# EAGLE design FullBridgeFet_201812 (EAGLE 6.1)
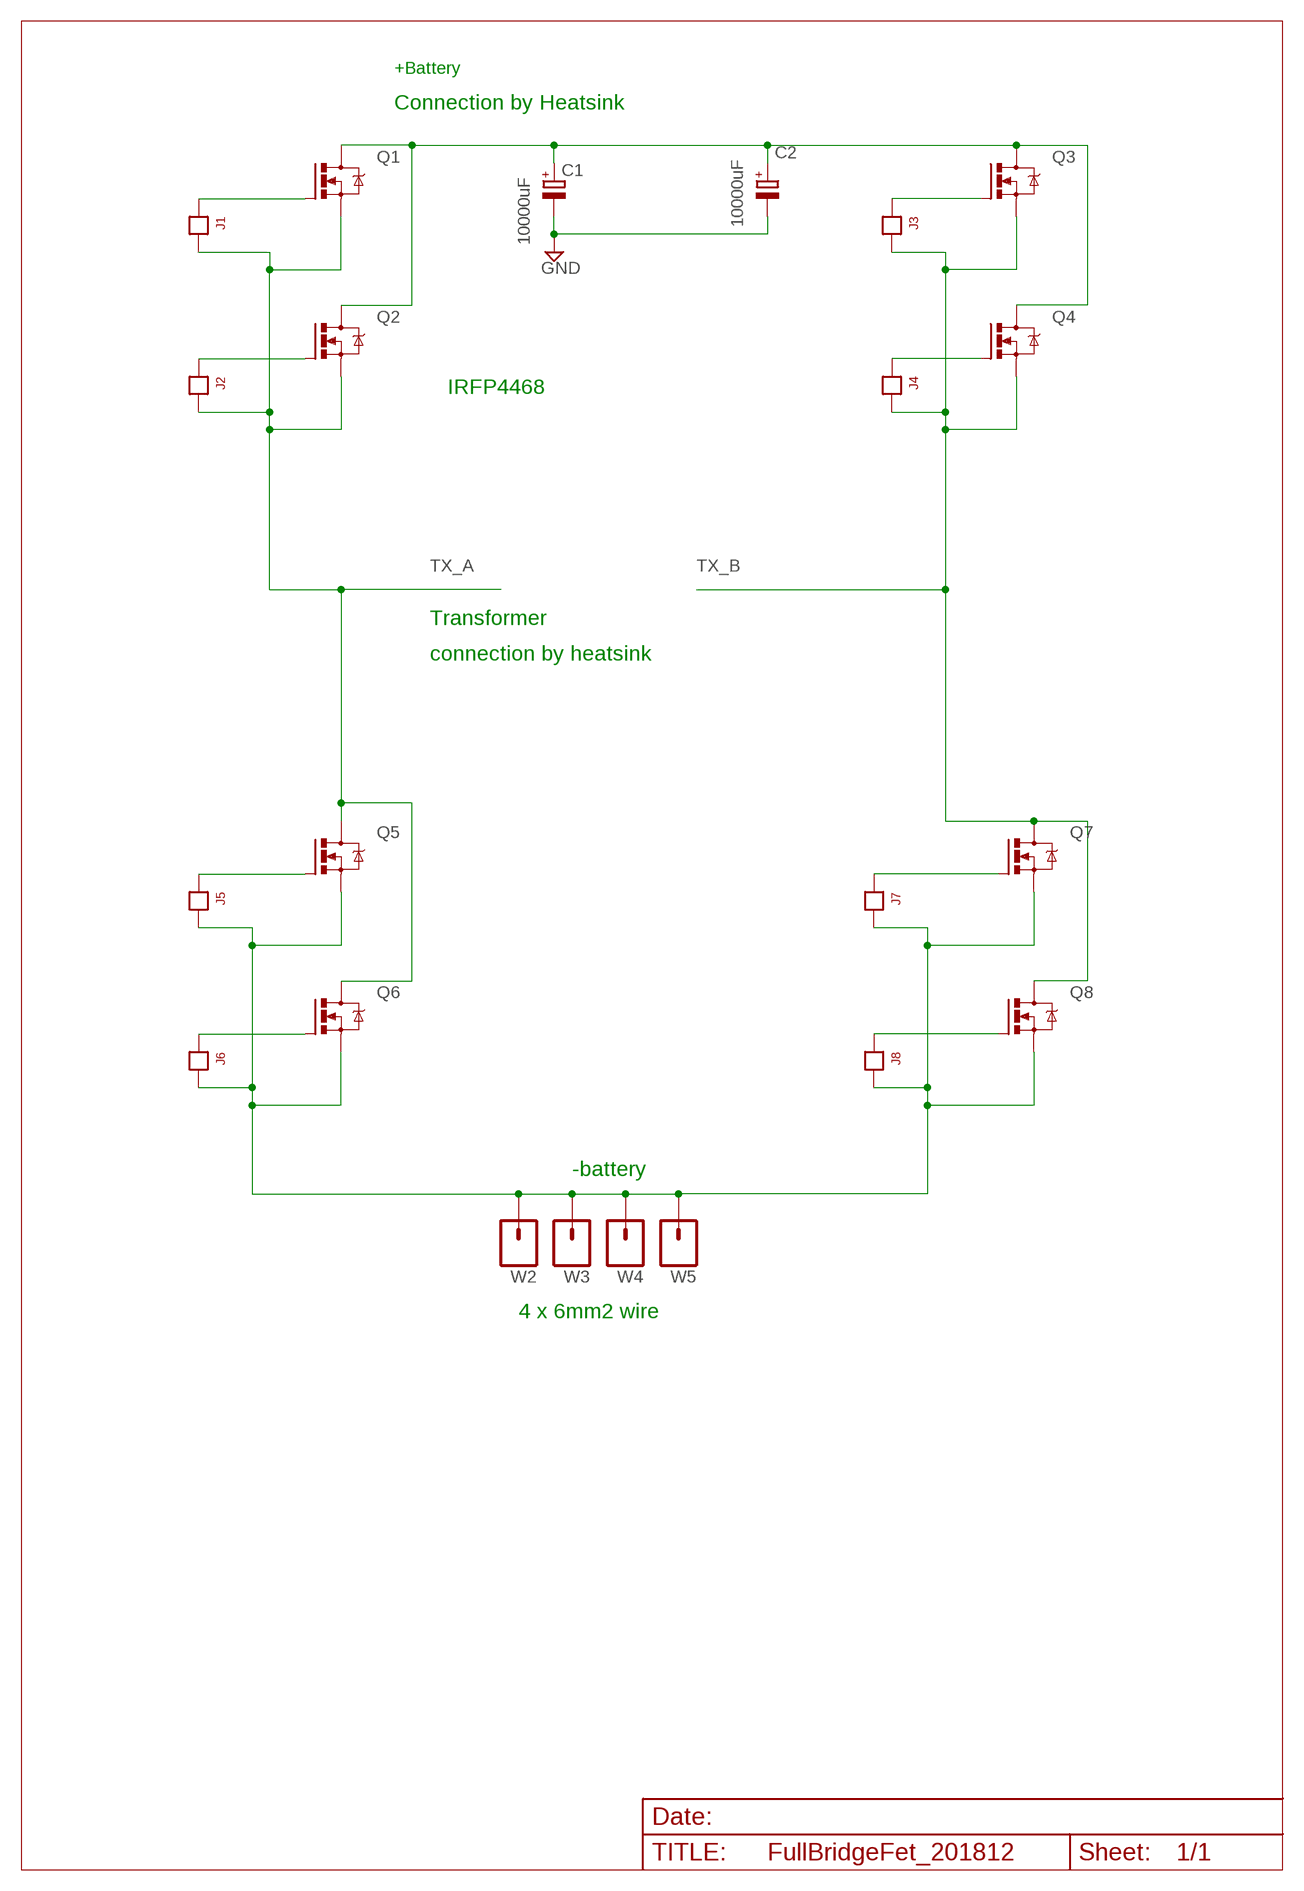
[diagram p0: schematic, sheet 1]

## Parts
C1  10000uF  C-RB3500LARGEPTH  [EB35D_LARGETH]
C2  10000uF  C-RB3500LARGEPTH  [EB35D_LARGETH]
J1  JP1  [JP1]
J2  JP1  [JP1]
J3  JP1  [JP1]
J4  JP1  [JP1]
J5  JP1  [JP1]
J6  JP1  [JP1]
J7  JP1  [JP1]
J8  JP1  [JP1]
Q1  IRFP4468  MOSFET-NCH-BIG  [TO247-WIRED]
Q2  MOSFET-NCH-BIG  [TO247-WIRED]
Q3  MOSFET-NCH-BIG  [TO247-WIRED]
Q4  MOSFET-NCH-BIG  [TO247-WIRED]
Q5  MOSFET-NCH-BIG  [TO247-WIRED]
Q6  MOSFET-NCH-BIG  [TO247-WIRED]
Q7  MOSFET-NCH-BIG  [TO247-WIRED]
Q8  MOSFET-NCH-BIG  [TO247-WIRED]
W2  M014MM2-WIREHOLE  [3.5MMWIREHOLE]
W3  M014MM2-WIREHOLE  [3.5MMWIREHOLE]
W4  M014MM2-WIREHOLE  [3.5MMWIREHOLE]
W5  M014MM2-WIREHOLE  [3.5MMWIREHOLE]

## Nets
+BATT: C1.+ C2.+ Q1.D Q1.DW(D) Q2.D Q2.DW(D) Q3.D Q3.DW(D) Q4.D Q4.DW(D)
GND: C1.- C2.- J5.2 J6.2 J7.2 J8.2 Q5.S Q5.SW(S) Q6.S Q6.SW(S) Q7.S Q7.SW(S) Q8.S Q8.SW(S) W2.P$1 W3.P$1 W4.P$1 W5.P$1
N$1: J1.1 Q1.G
N$2: J5.1 Q5.G
N$3: J6.1 Q6.G
N$4: J7.1 Q7.G
N$5: J2.1 Q2.G
N$6: J8.1 Q8.G
N$7: J3.1 Q3.G
N$10: J4.1 Q4.G
TX_A: J1.2 J2.2 Q1.S Q1.SW(S) Q2.S Q2.SW(S) Q5.D Q5.DW(D) Q6.D Q6.DW(D)
TX_B: J3.2 J4.2 Q3.S Q3.SW(S) Q4.S Q4.SW(S) Q7.D Q7.DW(D) Q8.D Q8.DW(D)

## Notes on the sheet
- +Battery
- Connection by Heatsink
- IRFP4468
- Transformer
- connection by heatsink
- -battery
- 4 x 6mm2 wire

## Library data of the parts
C1 C2 = Andrew Passive:C-RB3500
J1-J8 = Andrew Connectors:JP1
Q1-Q8 = Andrew Transistor:MOSFET-NCH-BIG
W2-W5 = Andrew:M01: Header 1

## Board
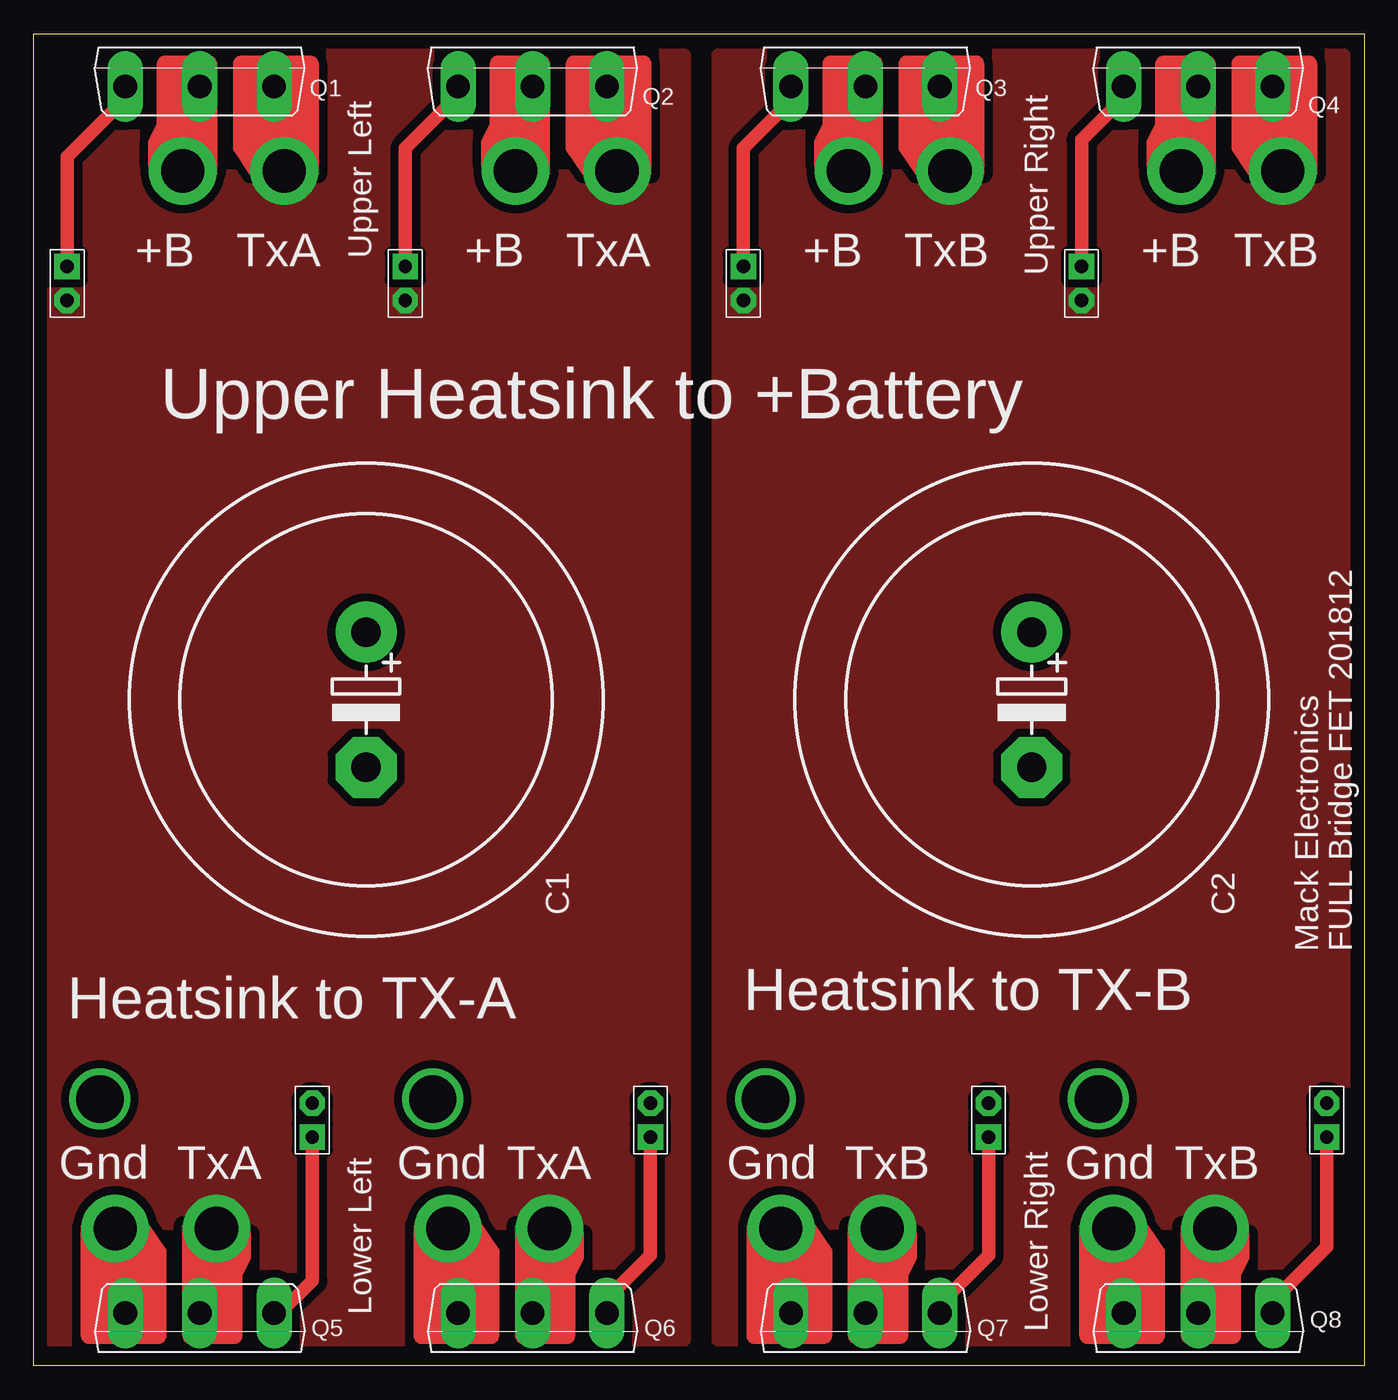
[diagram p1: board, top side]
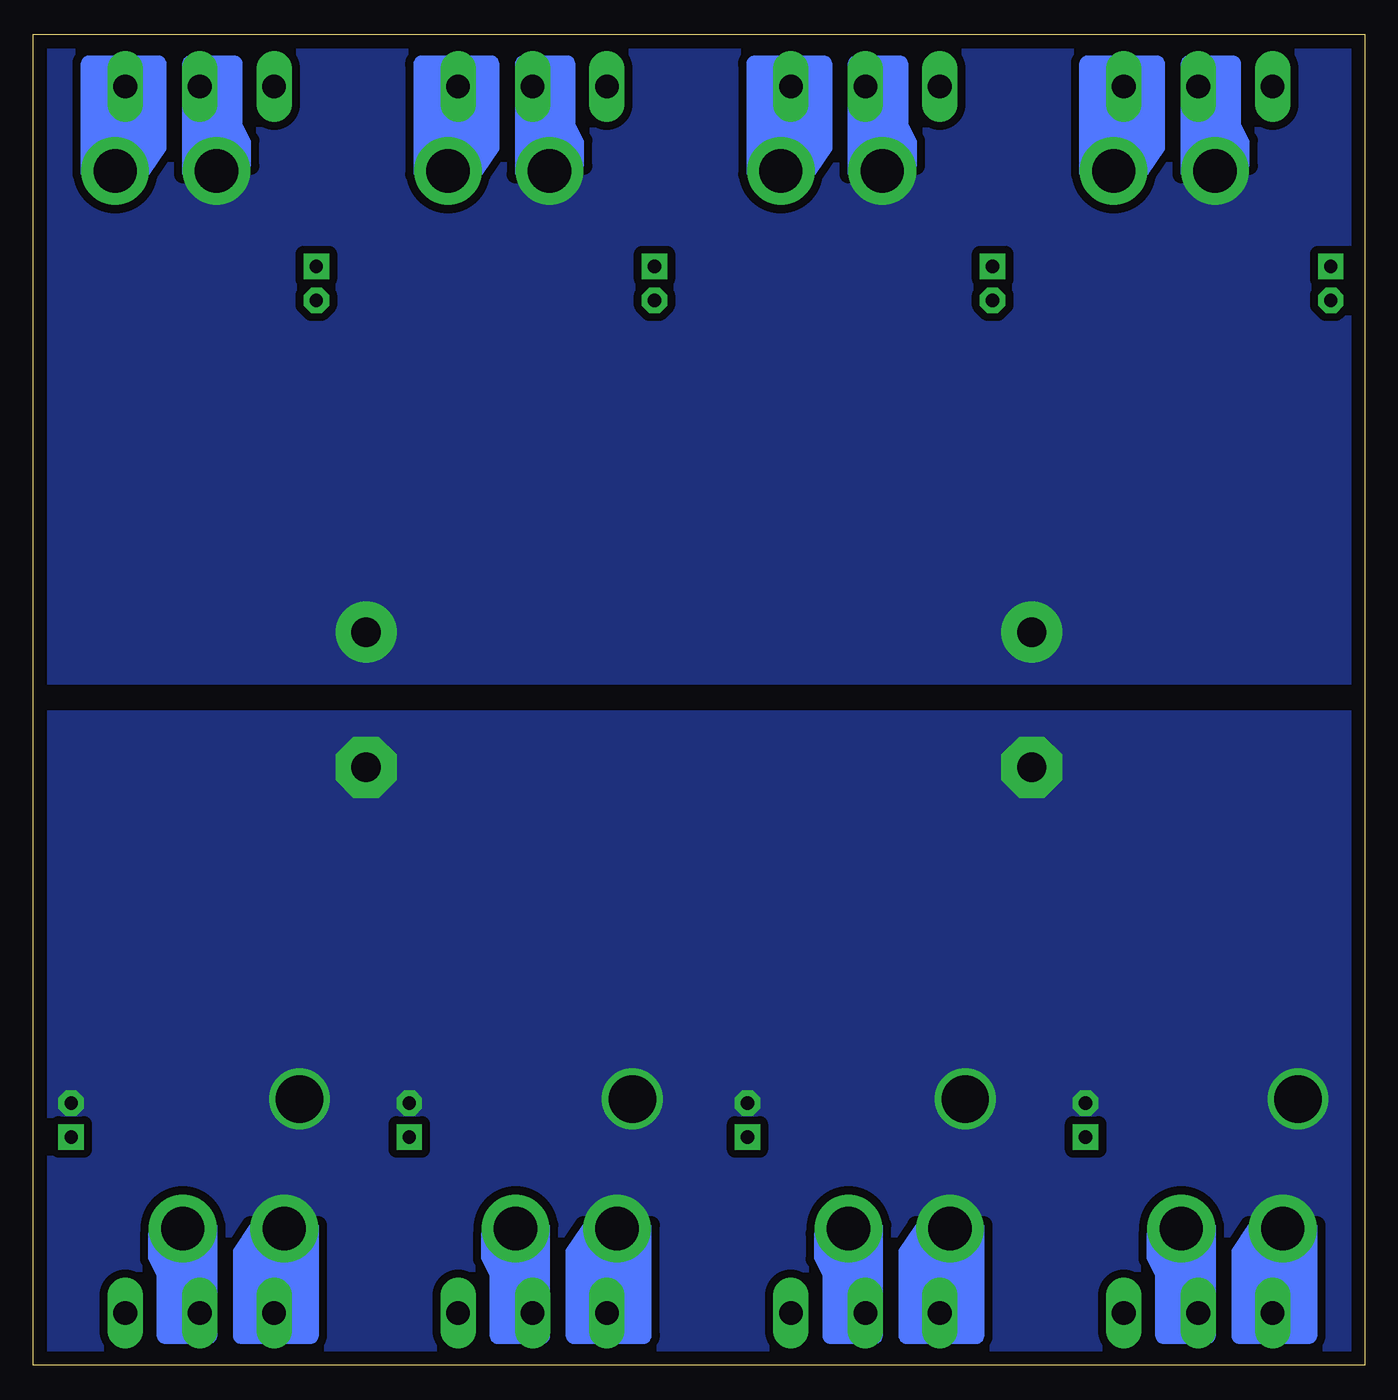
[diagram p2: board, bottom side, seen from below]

Size 100 x 100 mm. Coordinates in mm from the lower left corner, seen from the top.
Outline: 0,0 100,0 100,100 0,100 0,0
Copper layers (1*16): Top 0.035mm / dielectric 1.5mm / Bottom 0.035mm
Design rules: minimum track width 10mil, minimum drill 24mil, track to track 8mil, track to pad 8mil, pad to pad 8mil, via to via 8mil, smd to smd 8mil, copper to edge 40mil, drill to drill 8mil, minimum pad ring 10mil, minimum via ring 8mil, stop-mask expansion 4mil, vias tented up to drill 0mil, thermal gap 10mil

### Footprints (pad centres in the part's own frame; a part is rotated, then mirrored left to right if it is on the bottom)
EB35D_LARGETH = drill 2.2 pad 4.597: + -5.08,0 | drill 2.2 pad 4.597 octagon: - 5.08,0
JP1 = drill 1 pad 1.905 square: 1 -1.27,0 | drill 1 pad 1.905 octagon: 2 1.27,0
TO247-WIRED = drill 1.778 long: D 0,-2.921; G -5.588,-2.921; S 5.588,-2.921 | drill 3.25 pad 5.08: DW -1.27,-9.271; SW 6.35,-9.271
3.5MMWIREHOLE = drill 3.556: P$1 0,0

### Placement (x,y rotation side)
C1  25,50 270 top
C2  75,50 270 top
J1  2.54,81.28 270 top
J2  27.94,81.28 270 top
J3  53.34,81.28 270 top
J4  78.74,81.28 270 top
J5  20.95,18.41 90 top
J6  46.35,18.41 90 top
J7  71.75,18.41 90 top
J8  97.16,18.41 90 top
Q1  12.5,99 0 top
Q2  37.5,99 0 top
Q3  62.5,99 0 top
Q4  87.5,99 0 top
Q5  12.5,1 180 top
Q6  37.5,1 180 top
Q7  62.5,1 180 top
Q8  87.5,1 180 top
W2  80,20 0 top
W3  55,20 0 top
W4  30,20 0 top
W5  5,20 0 top

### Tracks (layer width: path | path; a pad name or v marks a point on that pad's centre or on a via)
+BATT
  pour Bottom (isolate 0.61, no thermals): 0.64,52.07 0.64,99.06 99.06,99.06 99.06,51.44 0.64,51.44
GND
  pour Bottom (isolate 0.61, no thermals): 0.64,48.9 99.06,48.9 99.06,1.27 0.64,1.27
N$1
  Top 1.016: Q1.G 6.91,95.18 2.54,90.81 J1.1
N$2
  Top 1.016: Q5.G 18.53,3.92 20.95,6.35 J5.1
N$3
  Top 1.016: Q6.G 43.09,4.99 46.35,8.26 J6.1
N$4
  Top 1.016: Q7.G 68.09,4.59 71.75,8.26 J7.1
N$5
  Top 1.016: Q2.G 31.91,95.41 27.94,91.44 J2.1
N$6
  Top 1.016: Q8.G 93.09,4.82 97.16,8.89 J8.1
N$7
  Top 1.016: Q3.G 56.91,95.01 53.34,91.44 J3.1
N$10
  Top 1.016: Q4.G 81.91,95.25 78.74,92.08 J4.1
TX_A
  pour Top (isolate 0.61, no thermals): 1.27,98.42 48.26,98.42 48.9,98.42 48.9,1.91 1.27,1.91
TX_B
  pour Top (isolate 0.61, no thermals): 51.44,98.42 98.42,98.42 98.42,1.91 51.44,1.91

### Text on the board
tPlace: +B | TxA | Upper Left | +B | TxA | +B | TxB | +B | TxB | Upper Right | Upper Heatsink to +Battery | Mack Electronics | FULL Bridge FET 201812 | Heatsink to TX-B | Heatsink to TX-A | Gnd | TxA | Gnd | TxA | Gnd | TxB | Gnd | TxB | Lower Left | Lower Right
